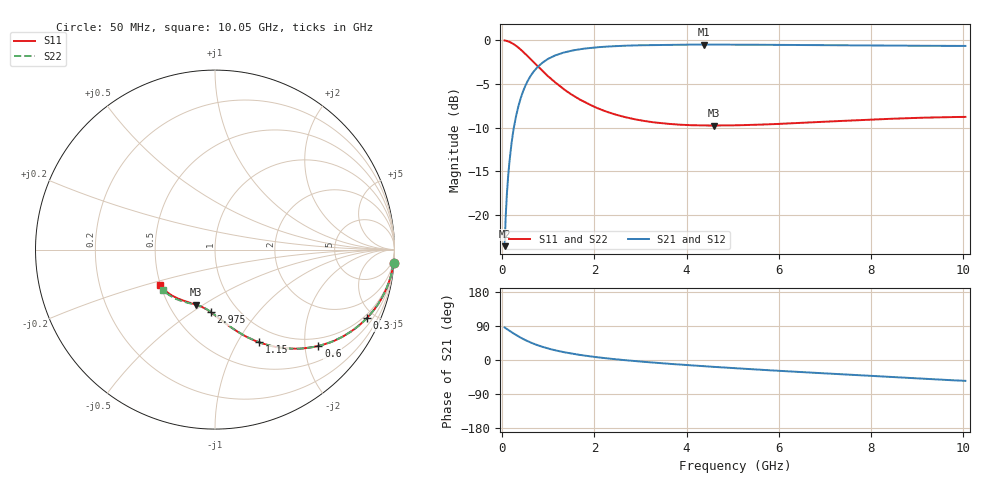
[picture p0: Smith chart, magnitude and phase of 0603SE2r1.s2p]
! AVX Thin Film Operation		Date: August 2001
! Description: Accu-P® Series, Thin Film, SMD, RF Capacitor
! Part Number: 06035J2R1ABT
! 50 MHz  -  10.05 GHz
! Serial Measurements
# mhz S db R 50
!	S11		S21		S12		S22
!	dB	Phase	dB	Phase	dB	Phase	dB	Phase
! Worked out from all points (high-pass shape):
!   401 points, 50 MHz to 10.05 GHz, reference 50 ohm
!   highest |S21| = -0.50 dB at 4.375 GHz (marker M1); lowest = -23.6 dB at 50 MHz (marker M2)
!   |S21| within 3 dB of the highest: 694.3 MHz to end of sweep
!   lowest |S11| = -9.8 dB at 4.6 GHz (marker M3), VSWR 1.96, Z = 34 - j23.4 ohm
!   |S11| at or under -10 dB: nowhere
!   |S22| runs from -9.8 to 0.0 dB; largest |S21 - S12| = 0
!   S11 on the Smith chart (normalised r, x): 50 MHz: 1, -27; 300 MHz: 0.82, -4.54; 600 MHz: 0.81, -2.29; 1.15 GHz: 0.81, -1.24; 2.975 GHz: 0.75, -0.59; 10.05 GHz: 0.50, -0.22
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50  -0.02 -4.2  -23.60 85.8  -23.60 85.8  -0.02 -4.2
75  -0.04 -6.3  -20.06 83.7  -20.06 83.7  -0.04 -6.3
125  -0.12 -10.5  -15.72 79.5  -15.72 79.5  -0.12 -10.5
175  -0.23 -14.4  -12.95 75.6  -12.95 75.6  -0.23 -14.4
225  -0.37 -18.5  -10.86 71.5  -10.86 71.5  -0.37 -18.5
300  -0.64 -24.1  -8.65 65.9  -8.65 65.9  -0.64 -24.1
425  -1.19 -32.7  -6.23 57.3  -6.23 57.3  -1.19 -32.7
600  -2.08 -43.0  -4.21 47.0  -4.21 47.0  -2.08 -43.0
725  -2.74 -49.1  -3.30 40.9  -3.30 40.9  -2.74 -49.1
875  -3.52 -55.4  -2.56 34.6  -2.56 34.6  -3.52 -55.3
1150  -4.84 -64.5  -1.73 25.5  -1.73 25.5  -4.84 -64.5
1375  -5.75 -70.2  -1.35 19.8  -1.35 19.8  -5.74 -70.1
1725  -6.91 -77.2  -1.00 12.7  -1.00 12.7  -6.91 -77.1
2250  -8.16 -85.4  -0.73 4.6  -0.73 4.6  -8.15 -85.1
2975  -9.15 -94.0  -0.57 -3.8  -0.57 -3.8  -9.14 -93.3
3400  -9.48 -98.3  -0.53 -8.0  -0.53 -8.0  -9.47 -97.5
4375  -9.77 -107.0  -0.50 -16.3  -0.50 -16.3  -9.75 -105.2
4600  -9.77 -108.8  -0.50 -18.2  -0.50 -18.2  -9.76 -106.8
5050  -9.75 -112.0  -0.50 -21.6  -0.50 -21.6  -9.73 -110.0
6725  -9.41 -125.0  -0.55 -33.4  -0.55 -33.4  -9.38 -122.0
8400  -9.01 -136.2  -0.61 -44.6  -0.61 -44.6  -8.98 -132.1
10050  -8.78 -147.6  -0.65 -55.0  -0.65 -55.0  -8.74 -141.8
